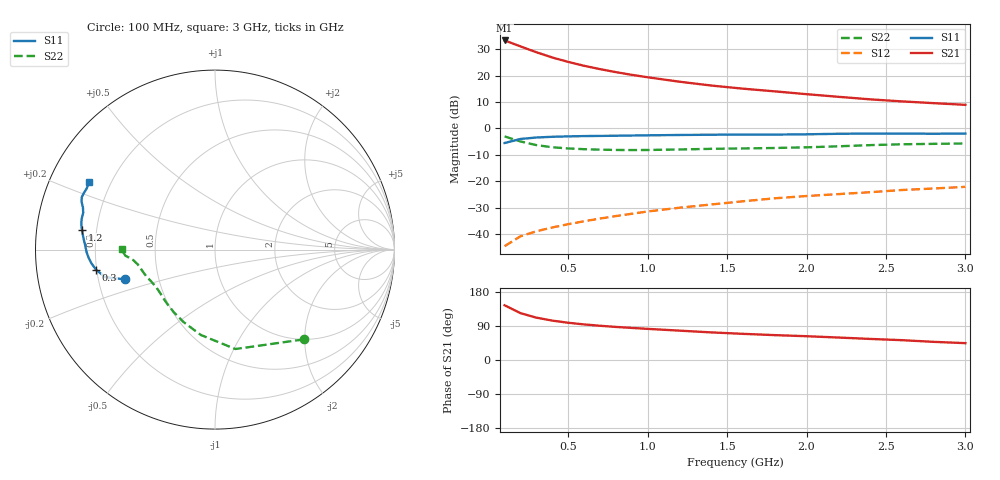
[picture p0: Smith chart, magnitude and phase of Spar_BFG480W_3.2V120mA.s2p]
! Filename: 3_2120BFG480.001
! Title: BFG480W
! Bias: Vce=3.2V; Ic=120mA
! Company: NXP Semiconductors NL
! User: Quality&Reliability T&D
! Measure time: 10 Nov 1999 / 11:58:23
#  MHz  S  MA  R 50
! Freq  S11  S21  S12  S22  :
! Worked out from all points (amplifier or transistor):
!   20 points, 100 MHz to 3 GHz, reference 50 ohm
!   highest |S21| = 33.3 dB at 100 MHz (marker M1)
!   |S21| within 3 dB of that: start of sweep to 233.8 MHz
!   unconditionally stable (mu >= 1): 592.6 MHz to end of sweep
!   at 400 MHz: K = 0.89, MSG = 32.2 dB, |S12| = -37.5 dB
!   at 1.2 GHz: K = 1.10, MAG = 22.0 dB, |S12| = -30.0 dB
!   at 3 GHz: K = 1.07, MAG = 14.0 dB, |S12| = -22.1 dB
!   S11 on the Smith chart (normalised r, x): 100 MHz: 0.32, -0.15; 300 MHz: 0.20, -0.08; 1.2 GHz: 0.14, +0.07; 3 GHz: 0.12, +0.25
100  0.5283 -161.7  46.1 144.3  0.005898 68.3  0.7034 -45.4
200  0.6305 -165.9  35.58 123.6  0.009073 61.4  0.5654 -78.4
300  0.6715 -170.3  27.58 111.8  0.01127 61.4  0.4821 -99.4
400  0.693 -173.7  21.94 103.9  0.01333 63.4  0.4397 -113.6
500  0.7055 -176.3  18.11 98.3  0.01535 65.7  0.417 -123.6
600  0.7146 -178.6  15.29 93.9  0.01746 67.6  0.4038 -130.8
700  0.7198 179.5  13.22 90.4  0.01964 69.5  0.3955 -136.4
800  0.7253 177.6  11.6 87.3  0.0219 71.1  0.3902 -141.0
900  0.7322 175.9  10.31 84.7  0.0242 72.7  0.3887 -145.0
1000  0.7385 174.3  9.269 82.2  0.02673 73.5  0.3899 -148.5
1200  0.7498 171.5  7.646 77.5  0.03151 74.8  0.3987 -154.2
1400  0.758 169.3  6.467 72.9  0.03627 75.5  0.4099 -158.3
1600  0.7626 167.0  5.64 69.0  0.04169 76.0  0.417 -161.6
1800  0.7622 164.4  5.016 65.6  0.0475 76.3  0.4253 -165.1
2000  0.7723 162.3  4.438 62.8  0.05243 76.8  0.438 -169.1
2200  0.7899 160.3  3.958 59.3  0.05697 76.6  0.4578 -172.5
2400  0.7976 158.5  3.544 55.6  0.0619 75.9  0.4816 -174.7
2600  0.7961 156.8  3.239 52.3  0.06816 75.1  0.5002 -176.1
2800  0.7917 154.5  3.001 47.9  0.07282 73.6  0.5094 -177.9
3000  0.7964 151.8  2.787 44.5  0.07824 72.8  0.5173 179.3
